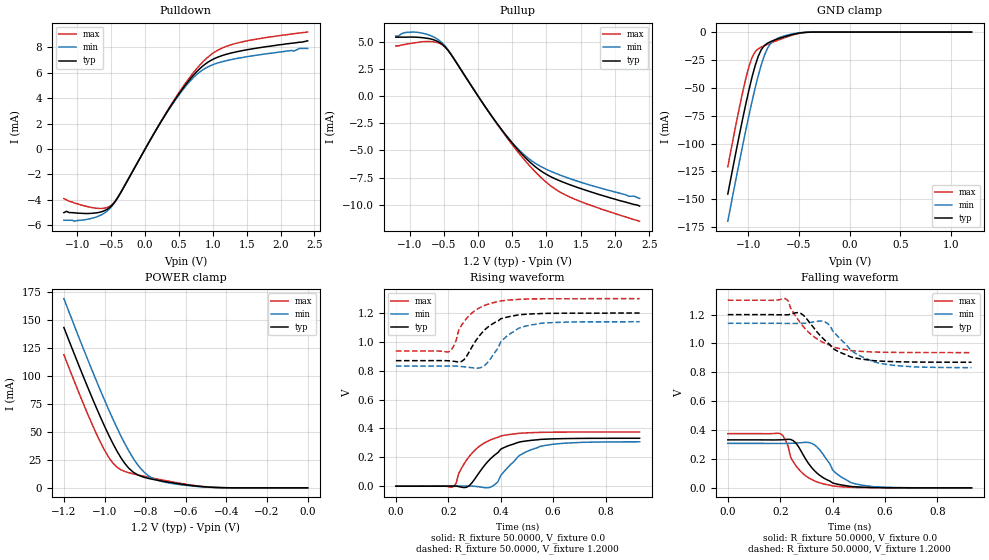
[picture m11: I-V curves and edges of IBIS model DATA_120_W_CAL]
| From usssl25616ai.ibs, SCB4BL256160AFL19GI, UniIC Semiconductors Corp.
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|   Model DATA_120_W_CAL
[Model]  DATA_120_W_CAL
Model_type I/O
Polarity   Non-Inverting
Enable   Active-High
Vinl =   0.3800V
Vinh =   0.8200V
Vmeas =  0.6000V
Cref =   5.0000pF
Rref =   50.0000
Vref =   0.6000V
C_comp   1.7430pF   1.7110pF   1.7640pF
[Temperature Range]   25.0000   85.0000   -40.0000
[Voltage Range]   1.2000V   1.1400V   1.3000V
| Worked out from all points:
|   slope of the pulldown table from 0 to 0.18 V, typ, clamps not added: 108 ohm
|   slope of the pullup table from 0 to 0.18 V, typ, clamps not added: 108 ohm
|   GND clamp passes 1 mA (typ) near -0.50 V on its own axis
|   POWER clamp passes 1 mA (typ) near -0.51 V on its own axis
|   rising waveform, R_fixture 50.0000, V_fixture 0.0: 20-80 % time 103ps typ, 110ps min, 101ps max; typ from 0 V to 0.332 V
|   rising waveform, R_fixture 50.0000, V_fixture 1.2000: 20-80 % time 96ps typ, 90.1ps min, 80.3ps max; typ from 0.87 V to 1.2 V
|   falling waveform, R_fixture 50.0000, V_fixture 0.0: 20-80 % time 91.6ps typ, 88.1ps min, 76.6ps max; typ from 0.332 V to 0 V
|   falling waveform, R_fixture 50.0000, V_fixture 1.2000: 20-80 % time 115ps typ, 125ps min, 116ps max; typ from 1.2 V to 0.87 V
[Pulldown]
|Voltage   I(typ)   I(min)   I(max)
-1.2V     -5mA       -5.6mA     -3.9mA
-1.04V    -5.02mA    -5.68mA    -4.25mA
-760mV    -5.043mA   -5.406mA   -4.623mA
-600mV    -4.846mA   -5.03mA    -4.649mA
-480mV    -4.371mA   -4.42mA    -4.339mA
-360mV    -3.417mA   -3.408mA   -3.43mA
360mV     3.218mA    3.175mA    3.277mA
640mV     5.334mA    5.197mA    5.495mA
840mV     6.469mA    6.181mA    6.777mA
1.04V     7.144mA    6.701mA    7.66mA
1.28V     7.554mA    7.034mA    8.209mA
2.4V      8.5mA      7.9mA      9.19mA
[Pullup]
|Voltage   I(typ)   I(min)   I(max)
-1.2V     5.4mA      5.5mA      4.6mA
-1.08V    5.4mA      5.8mA      4.72mA
-880mV    5.39mA     5.84mA     4.92mA
-680mV    5.219mA    5.508mA    4.989mA
-520mV    4.73mA     4.853mA    4.698mA
-400mV    3.86mA     3.907mA    3.883mA
320mV     -2.881mA   -2.893mA   -2.942mA
560mV     -4.768mA   -4.697mA   -4.953mA
760mV     -6.076mA   -5.84mA    -6.448mA
1.04V     -7.336mA   -6.848mA   -8.14mA
1.28V     -8mA       -7.45mA    -9.095mA
2.36V     -10.1mA    -9.4mA     -11.5mA
[GND_clamp]
|Voltage   I(typ)   I(min)   I(max)
-1.2V     -145.3mA   -169.7mA   -120.8mA
-1.11V    -103.1mA   -127.3mA   -78.51mA
-1.05V    -76.2mA    -100.1mA   -52.43mA
-990mV    -51.2mA    -74mA      -30.39mA
-960mV    -39.9mA    -61.63mA   -22.48mA
-900mV    -21.67mA   -39mA      -15mA
-870mV    -15.78mA   -29.25mA   -13.45mA
-810mV    -10.04mA   -14.72mA   -11.07mA
-750mV    -7.557mA   -7.71mA    -8.865mA
-600mV    -3.111mA   -2.463mA   -3.804mA
-420mV    -215.4uA   -156.1uA   -235uA
1.2V      1.597nA    5.589nA    1.463nA
[POWER_clamp]
|Voltage   I(typ)   I(min)   I(max)
-1.2V     143mA      168.8mA    118.7mA
-1.06V    79.88mA    104.3mA    56.26mA
-1.02V    63.08mA    86.79mA    40.63mA
-980mV    47.32mA    69.97mA    27.48mA
-940mV    33.2mA     54.05mA    18.67mA
-880mV    17.43mA    32.78mA    13.45mA
-840mV    11.87mA    21.34mA    11.69mA
-800mV    9.133mA    13.1mA     10.12mA
-720mV    6.135mA    5.731mA    7.166mA
-560mV    1.838mA    1.456mA    2.161mA
-420mV    156.9uA    132.7uA    153uA
0V        1.597nA    1.927nA    2.16nA
[Ramp]
| variable   typ   min   max
dV/dt_r  0.1993/0.1052n   0.1846/0.1146n   0.2253/95.2293p
dV/dt_f  0.1979/0.1159n   0.1844/0.1254n   0.2179/0.1078n
R_load = 50.0000
[Rising Waveform]
R_fixture= 50.0000
V_fixture= 0.0
V_fixture_min= 0.0
V_fixture_max= 0.0
|time   V(typ)   V(min)   V(max)
0s        0V         0V         0V
220ps     1.212mV    192.7uV    -2.406mV
250ps     -6.397mV   820.6uV    122.7mV
290ps     22.9mV     787.2uV    228.1mV
360ps     188.1mV    -7.66mV    320mV
390ps     233.7mV    32.6mV     339.1mV
400ps     256.1mV    74mV       348.1mV
470ps     305.5mV    210.9mV    366.7mV
550ps     324.1mV    275.6mV    373mV
930ps     332.2mV    307.6mV    375.5mV
[Rising Waveform]
R_fixture= 50.0000
V_fixture= 1.2000
V_fixture_min= 1.1400
V_fixture_max= 1.3000
|time   V(typ)   V(min)   V(max)
0s        870mV      832.3mV    936.9mV
200ps     869.1mV    832.9mV    930.2mV
220ps     865.7mV    832.8mV    969mV
250ps     863.8mV    829.2mV    1.114V
330ps     1.066V     826.1mV    1.246V
360ps     1.115V     880.1mV    1.266V
400ps     1.16V      1V         1.284V
470ps     1.188V     1.096V     1.295V
550ps     1.196V     1.128V     1.298V
930ps     1.2V       1.14V      1.3V
[Falling Waveform]
R_fixture= 50.0000
V_fixture= 0.0
V_fixture_min= 0.0
V_fixture_max= 0.0
|time   V(typ)   V(min)   V(max)
0s        332.3mV    307.8mV    375.5mV
200ps     332.6mV    307.4mV    376.1mV
220ps     334.6mV    307.4mV    330.4mV
240ps     335.1mV    308.5mV    211.1mV
280ps     253.3mV    313mV      110.4mV
330ps     120mV      298.6mV    48.67mV
400ps     33.77mV    123.2mV    13.1mV
470ps     9.429mV    36.23mV    3.526mV
550ps     2.241mV    8.938mV    805uV
930ps     3.658uV    17.3uV     1.051uV
[Falling Waveform]
R_fixture= 50.0000
V_fixture= 1.2000
V_fixture_min= 1.1400
V_fixture_max= 1.3000
|time   V(typ)   V(min)   V(max)
0s        1.2V       1.14V      1.3V
220ps     1.199V     1.139V     1.311V
280ps     1.207V     1.139V     1.135V
320ps     1.127V     1.147V     1.059V
370ps     1.023V     1.15V      1.002V
420ps     945.9mV    1.049V     967.4mV
480ps     902.4mV    939.9mV    949.3mV
570ps     879.4mV    866.8mV    940.3mV
710ps     871.5mV    838.2mV    937.4mV
930ps     870.1mV    832.7mV    936.9mV
